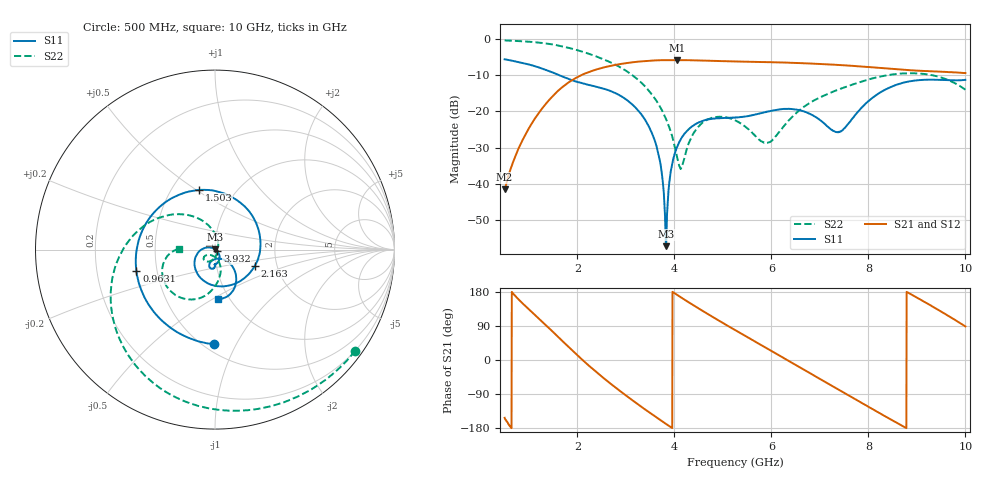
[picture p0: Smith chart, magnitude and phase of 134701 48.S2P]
!  2-Port S-parameters saved by WinCal
! VAR MeasName=S-Parameters (CALIBRATED_DATA) read from VNA (N5242A)
! VAR MeasDate=2013-7-3 16:38:31
! VAR NAME=134701 48
! VAR FILENAME=134701 48.S2P
! VAR DATE=2013-7-3 16:38:31
! VAR PHYS_PORTS=1,2
# Hz S MA R 50
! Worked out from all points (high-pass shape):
!   1601 points, 500 MHz to 10 GHz, reference 50 ohm
!   highest |S21| = -5.75 dB at 4.051 GHz (marker M1); lowest = -41.5 dB at 500 MHz (marker M2)
!   |S21| within 3 dB of the highest: 2.303 GHz to 9.123 GHz (6.82 GHz wide, 119 % of centre)
!   lowest |S11| = -57.3 dB at 3.831 GHz (marker M3), VSWR 1.00, Z = 50.1 + j0.0888 ohm
!   |S11| at or under -10 dB: 1.633 GHz to end of sweep
!   |S22| runs from -35.9 to -0.3 dB; largest |S21 - S12| = 0.0026
!   S11 on the Smith chart (normalised r, x): 500 MHz: 0.56, -0.82; 963.1 MHz: 0.38, -0.12; 1.503 GHz: 0.68, +0.51; 2.163 GHz: 1.54, -0.29; 3.932 GHz: 1.02, -0.02; 10 GHz: 0.89, -0.53
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5e8  0.5277 -90.5  0.008369 -152.6  0.008407 -152.9  0.9631 -35.9
9.63125e8  0.4542 -164.6  0.05288 138.4  0.0529 138.0  0.9287 -68.6
1.503438e9  0.3441 104.9  0.1664 73.5  0.1661 73.3  0.8446 -107.3
2.085312e9  0.2481 -7.2  0.3194 2.5  0.3191 2.5  0.6791 -147.4
2.1625e9  0.24 -21.7  0.3365 -6.4  0.336 -6.5  0.6541 -152.5
2.554375e9  0.2055 -84.4  0.409 -49.1  0.4087 -49.0  0.5235 -178.0
3.16e9  0.1203 -156.5  0.4821 -108.6  0.4818 -108.5  0.3086 140.7
3.46875e9  0.06295 173.4  0.5037 -137.0  0.5034 -137.0  0.1957 118.0
3.670625e9  0.026 154.6  0.5122 -155.1  0.5113 -155.0  0.1271 101.8
3.830938e9  0.001361 40.6  0.5149 -169.0  0.5149 -169.0  0.07795 86.2
3.931875e9  0.01555 -37.8  0.5153 -177.7  0.5156 -177.7  0.05078 72.8
4.050625e9  0.03154 -47.4  0.5157 172.4  0.5155 172.3  0.02422 41.4
4.151562e9  0.04363 -55.0  0.515 164.1  0.5147 164.0  0.01676 -27.9
4.37125e9  0.06275 -68.3  0.5114 146.2  0.5119 146.2  0.04686 -93.5
4.638438e9  0.07618 -80.6  0.5057 125.3  0.5056 125.3  0.07434 -117.1
5.25e9  0.08234 -91.4  0.4931 79.1  0.4934 79.1  0.07551 -145.1
5.926875e9  0.1 -91.9  0.4819 29.3  0.482 29.3  0.037 -108.8
6.835312e9  0.0897 -110.8  0.4608 -37.7  0.4606 -37.7  0.1371 -77.3
7.41125e9  0.05222 -73.2  0.4398 -80.2  0.4396 -80.2  0.2044 -89.8
8.420625e9  0.2118 -56.2  0.3925 -154.0  0.3915 -154.0  0.3199 -120.7
9.145e9  0.2744 -79.6  0.3638 154.1  0.3643 154.2  0.3314 -150.5
1e10  0.2742 -86.1  0.3407 88.6  0.3414 88.7  0.2001 178.9
